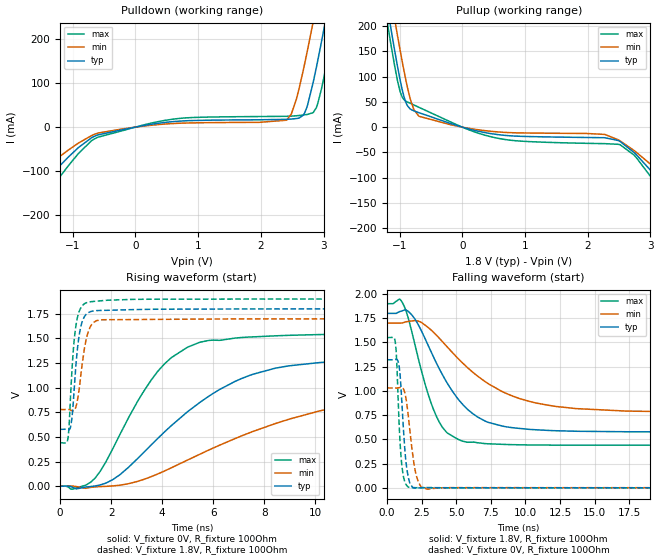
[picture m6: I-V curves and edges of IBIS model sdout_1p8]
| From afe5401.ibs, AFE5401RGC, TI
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|   sdout_1p8 Model
[Model]   sdout_1p8
Model_type   Output
Polarity   Non-Inverting
Vmeas = 0.9
Vref = 0
Cref = 5pF
Rref = 100
|   typ   min   max
|   (nom PVT)   (fast PVT)   (slow PVT)
C_comp   1.609e-12   1.569e-12   1.659e-12
| Where nom  PVT is Nominal Process, 1.8V, 27C
|   Fast PVT is Strong Process,  1.9V, -40C
|   Slow PVT is Weak Process,   1.7V, 125C
[Voltage Range]   1.8   1.7   1.9
|Junction Temperature
[Temperature Range]   27   125   -40
[Pullup Reference]   1.8   1.7   1.9
[Pulldown Reference]   0   0   0
[Power Clamp Reference]   1.8   1.7   1.9
[GND Clamp Reference]   0   0   0
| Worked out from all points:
|   slope of the pulldown table from 0 to 0.27 V, typ, clamps not added: 39.5 ohm
|   slope of the pullup table from 0 to 0.27 V, typ, clamps not added: 31.9 ohm
|   falling waveform, V_fixture 1.8V, R_fixture 100Ohm: 20-80 % time 3.04ns typ, 4.85ns min, 1.79ns max; typ from 1.8 V to 0.577 V
|   rising waveform, V_fixture 0V, R_fixture 100Ohm: 20-80 % time 3.83ns typ, 6.74ns min, 2.16ns max; typ from 0 V to 1.32 V
|   rising waveform, V_fixture 1.8V, R_fixture 100Ohm: 20-80 % time 253ps typ, 311ps min, 231ps max; typ from 0.577 V to 1.8 V
|   falling waveform, V_fixture 0V, R_fixture 100Ohm: 20-80 % time 375ps typ, 532ps min, 300ps max; typ from 1.32 V to 0 V
[Pulldown]
|   Voltage   I(typ)   I(min)   I(max)
-1.8V     -234.3mA   -154.2mA   -314.1mA
-1.635V   -162.2mA   -116.9mA   -224.1mA
-1.54V    -140.2mA   -105mA     -182.1mA
-598.1mV  -17.51mA   -13.46mA   -22.87mA
682mV     13.43mA    8.736mA    19.52mA
2.409V    17.67mA    15.76mA    24.59mA
2.564V    19.45mA    62.17mA    25.8mA
2.675V    26.86mA    128.2mA    27.54mA
2.833V    100.7mA    238.3mA    32.81mA
2.996V    215.1mA    358.8mA    106.1mA
3.201V    372.1mA    516.6mA    258.6mA
3.6V      686.9mA    828.6mA    575.6mA
[Pullup]
|   Voltage   I(typ)   I(min)   I(max)
-1.8V     721mA      774.8mA    698.6mA
-1.186V   231.1mA    293.3mA    200mA
-1.142V   197.8mA    260.3mA    166.5mA
-1.076V   149.8mA    211.8mA    119.3mA
-990.8mV  92.91mA    151.7mA    70.14mA
-899.4mV  48.8mA     92.79mA    51.4mA
-691.6mV  28.54mA    21.49mA    39.21mA
574.2mV   -14.85mA   -9.506mA   -22.14mA
2.489V    -26.51mA   -25.16mA   -33.94mA
2.777V    -54.76mA   -49.88mA   -60.57mA
3.402V    -148.4mA   -121.8mA   -172.2mA
3.6V      -229.2mA   -187.4mA   -258.6mA
[Ramp]
R_load = 100
|   typ   min   max
dV/dt_r   0.792891/3.82752e-09   0.618152/6.70679e-09   0.930161/2.16273e-09
dV/dt_f   0.733821/3.03349e-09   0.553213/4.84941e-09   0.875843/1.79132e-09
[Falling Waveform]
V_fixture = 1.8V
V_fixture_min = 1.7V
V_fixture_max = 1.9V
R_fixture = 100Ohm
|   Time   V(typ)   V(min)   V(max)
0s        1.8V       1.7V       1.9V
960ps     1.82V      1.699V     1.942V
1.81ns    1.781V     1.722V     1.6V
2.75ns    1.539V     1.679V     1.071V
3.6ns     1.279V     1.571V     728.4mV
4.38ns    1.073V     1.449V     563.4mV
5.76ns    817.7mV    1.247V     471.4mV
10.32ns   602.6mV    890.9mV    442.3mV
17.29ns   578.5mV    791.7mV    440.2mV
75ns      577mV      778mV      440.3mV
[Rising Waveform]
V_fixture = 0V
V_fixture_min = 0V
V_fixture_max = 0V
R_fixture = 100Ohm
|   Time   V(typ)   V(min)   V(max)
0s        1.294nV    91.72nV    568pV
1.38ns    2.355mV    -6.935mV   85.74mV
3.27ns    340.9mV    68.02mV    961.5mV
4.35ns    613.3mV    185.8mV    1.304V
5.47ns    850mV      323.9mV    1.461V
7.12ns    1.094V     511.7mV    1.51V
8.92ns    1.22V      676mV      1.531V
12.92ns   1.293V     895.2mV    1.547V
20.53ns   1.318V     1.005V     1.55V
75ns      1.321V     1.03V      1.55V
[Rising Waveform]
V_fixture = 1.8V
V_fixture_min = 1.7V
V_fixture_max = 1.9V
R_fixture = 100Ohm
|   Time   V(typ)   V(min)   V(max)
0s        577mV      778mV      440.3mV
310ps     570.9mV    779.3mV    490.7mV
430ps     630.8mV    770.7mV    1.026V
530ps     910mV      767.4mV    1.424V
640ps     1.294V     827.7mV    1.664V
740ps     1.523V     976.8mV    1.771V
950ps     1.72V      1.396V     1.852V
1.11ns    1.763V     1.575V     1.869V
1.89ns    1.786V     1.691V     1.889V
75ns      1.8V       1.7V       1.9V
[Falling Waveform]
V_fixture = 0V
V_fixture_min = 0V
V_fixture_max = 0V
R_fixture = 100Ohm
|   Time   V(typ)   V(min)   V(max)
0s        1.321V     1.03V      1.55V
590ps     1.324V     1.03V      1.511V
700ps     1.325V     1.03V      1.302V
850ps     1.276V     1.032V     747.1mV
1.16ns    664.7mV    1.025V     138.4mV
1.41ns    218.6mV    886.4mV    26.93mV
1.74ns    28.59mV    477.4mV    1.415mV
2.23ns    -1.624mV   74.57mV    1.99mV
2.95ns    2.753mV    -13.85mV   959.5uV
75ns      -1.159nV   91.16nV    -1.112nV
